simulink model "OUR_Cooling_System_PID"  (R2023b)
settings: Solver=VariableStepAuto  StartTime=0.0  StopTime=10.0  RelTol=1e-3
undefined symbols (not defined in the file): area_air, area_fins, area_primary, cp_air, EM_Spd, EM_Trq, eta_inv, eta_mot, h_tube, HC_min, HC_nom, L_tube, n_tubes, P_nom_pump, rho_air, T_amb, Th_Loss_Inv, Th_Loss_Mot, time, Veh_Spd, vel_air_nom, w_radiator
libraries: fl_lib x29, nesl_utility x16, SimscapeFluids_lib x8, slpidlib x2

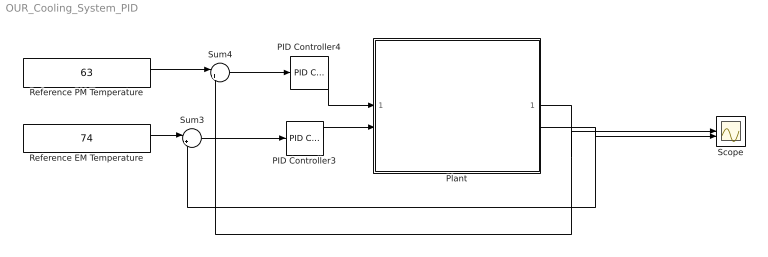
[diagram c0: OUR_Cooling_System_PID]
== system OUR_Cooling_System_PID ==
  PID Controller3 : slpidlib/PID Controller  Controller=PID  Form=Parallel  TimeDomain=Continuous-time  UseExternalTs=off  SampleTime=-1  IntegratorMethod=Forward Euler  FilterMethod=Forward Euler  ControllerParametersSource=internal  P=-0.153121737638524  I=-0.00104451455208141  UseKiTs=off  D=1.82506315689532  N=0.0838994185269757  UseFilter=on  TunerSelectOption=Transfer Function Based (PID Tuner App)  InitialConditionSource=internal  InitialConditionForIntegrator=0  InitialConditionForFilter=0  DifferentiatorICPrevScaledInput=0  ExternalReset=none  TrackingMode=off  Kt=1  LimitOutput=off  SatLimitsSource=internal  UpperSaturationLimit=inf  LowerSaturationLimit=-inf  LinearizeAsGain=on  AntiWindupMode=none  Kb=1  LimitIntegrator=off  UpperIntegratorSaturationLimit=inf  LowerIntegratorSaturationLimit=-inf  POutMin=[]  POutMax=[]  IOutMin=[]  IOutMax=[]  DOutMin=[]  DOutMax=[]  NOutMin=[]  NOutMax=[]  SumOutMin=[]  SumOutMax=[]  SaturationOutMin=[]  SaturationOutMax=[]  PParamMin=[]  PParamMax=[]  IParamMin=[]  IParamMax=[]  DParamMin=[]  DParamMax=[]  NParamMin=[]  NParamMax=[]  KbParamMin=[]  KbParamMax=[]  KtParamMin=[]  KtParamMax=[]  KbOutMin=[]  KbOutMax=[]  KtOutMin=[]  KtOutMax=[]  IntegratorOutMin=[]  IntegratorOutMax=[]  FilterOutMin=[]  FilterOutMax=[]  SumI1OutMin=[]  SumI1OutMax=[]  SumI2OutMin=[]  SumI2OutMax=[]  SumI3OutMin=[]  SumI3OutMax=[]  SumI4OutMin=[]  SumI4OutMax=[]  SumDOutMin=[]  SumDOutMax=[]  DifferentiatorOutMin=[]  DifferentiatorOutMax=[]  FilterDiffOutCoefMin=[]  FilterDiffOutCoefMax=[]  ReciprocalOutMin=[]  ReciprocalOutMax=[]  SumDenOutMin=[]  SumDenOutMax=[]  SumNumOutMin=[]  SumNumOutMax=[]  DivideOutMin=[]  DivideOutMax=[]  UdiffTsProdOutMin=[]  UdiffTsProdOutMax=[]  NTsProdOutMin=[]  NTsProdOutMax=[]  UintegralTsProdOutMin=[]  UintegralTsProdOutMax=[]  UngainTsProdOutMin=[]  UngainTsProdOutMax=[]  ClampingZeroOutDataTypeStr=Inherit: Inherit via back propagation  ClampingZeroOutMin=[]  ClampingZeroOutMax=[]  FilterDenConstantOutDataTypeStr=Inherit: Inherit via back propagation  FilterDenConstantOutMin=[]  FilterDenConstantOutMax=[]  PCopyOutDataTypeStr=Inherit: Inherit via back propagation  PCopyOutMin=[]  PCopyOutMax=[]  NCopyOutDataTypeStr=Inherit: Inherit via back propagation  NCopyOutMin=[]  NCopyOutMax=[]  IntegratorContinuousStateAttributes=''  IntegratorStateMustResolveToSignalObject=off  IntegratorRTWStateStorageClass=Auto  FilterContinuousStateAttributes=''  FilterStateMustResolveToSignalObject=off  FilterRTWStateStorageClass=Auto  ParallelPVariant=InternalParameters  IdealPVariant=Disabled  IVariant=InternalParameters  DVariant=InternalParameters  IntegratorVariant=Continuous  SatVariant=Disabled  AWVariant=Passthrough  PCopyVariant=Disabled  TRVariant=Disabled  FdbkBlocksVariant=Forward  IdealPFdbkVariant=Disabled  SatFdbkVariant=Disabled  DerivativeFilterVariant=ContFilter  NVariant=InternalParameters  NCopyVariant=Disabled  FilterICVariant=InternalICsFilter  IntegratorICVariant=InternalICs  ExternalResetVariant=Disabled  TRSumVariant=Passthrough  SumFdbkVariant=Disabled  SumVariant=Sum_PID  TsampFilterVariant=InternalTs  TsampNgainVariant=Passthrough  TsampIntegralVariant=Disabled_SignalSpec  ExternalSaturationOutDataTypeStr=Inherit: Same as second input
  PID Controller4 : slpidlib/PID Controller  Controller=PID  Form=Parallel  TimeDomain=Continuous-time  UseExternalTs=off  SampleTime=-1  IntegratorMethod=Forward Euler  FilterMethod=Forward Euler  ControllerParametersSource=internal  P=-0.690992720516584  I=-0.00856089702379571  UseKiTs=off  D=21.0718466167788  N=0.0327922242925958  UseFilter=on  TunerSelectOption=Transfer Function Based (PID Tuner App)  InitialConditionSource=internal  InitialConditionForIntegrator=0  InitialConditionForFilter=0  DifferentiatorICPrevScaledInput=0  ExternalReset=none  TrackingMode=off  Kt=1  LimitOutput=off  SatLimitsSource=internal  UpperSaturationLimit=inf  LowerSaturationLimit=-inf  LinearizeAsGain=on  AntiWindupMode=none  Kb=1  LimitIntegrator=off  UpperIntegratorSaturationLimit=inf  LowerIntegratorSaturationLimit=-inf  POutMin=[]  POutMax=[]  IOutMin=[]  IOutMax=[]  DOutMin=[]  DOutMax=[]  NOutMin=[]  NOutMax=[]  SumOutMin=[]  SumOutMax=[]  SaturationOutMin=[]  SaturationOutMax=[]  PParamMin=[]  PParamMax=[]  IParamMin=[]  IParamMax=[]  DParamMin=[]  DParamMax=[]  NParamMin=[]  NParamMax=[]  KbParamMin=[]  KbParamMax=[]  KtParamMin=[]  KtParamMax=[]  KbOutMin=[]  KbOutMax=[]  KtOutMin=[]  KtOutMax=[]  IntegratorOutMin=[]  IntegratorOutMax=[]  FilterOutMin=[]  FilterOutMax=[]  SumI1OutMin=[]  SumI1OutMax=[]  SumI2OutMin=[]  SumI2OutMax=[]  SumI3OutMin=[]  SumI3OutMax=[]  SumI4OutMin=[]  SumI4OutMax=[]  SumDOutMin=[]  SumDOutMax=[]  DifferentiatorOutMin=[]  DifferentiatorOutMax=[]  FilterDiffOutCoefMin=[]  FilterDiffOutCoefMax=[]  ReciprocalOutMin=[]  ReciprocalOutMax=[]  SumDenOutMin=[]  SumDenOutMax=[]  SumNumOutMin=[]  SumNumOutMax=[]  DivideOutMin=[]  DivideOutMax=[]  UdiffTsProdOutMin=[]  UdiffTsProdOutMax=[]  NTsProdOutMin=[]  NTsProdOutMax=[]  UintegralTsProdOutMin=[]  UintegralTsProdOutMax=[]  UngainTsProdOutMin=[]  UngainTsProdOutMax=[]  ClampingZeroOutDataTypeStr=Inherit: Inherit via back propagation  ClampingZeroOutMin=[]  ClampingZeroOutMax=[]  FilterDenConstantOutDataTypeStr=Inherit: Inherit via back propagation  FilterDenConstantOutMin=[]  FilterDenConstantOutMax=[]  PCopyOutDataTypeStr=Inherit: Inherit via back propagation  PCopyOutMin=[]  PCopyOutMax=[]  NCopyOutDataTypeStr=Inherit: Inherit via back propagation  NCopyOutMin=[]  NCopyOutMax=[]  IntegratorContinuousStateAttributes=''  IntegratorStateMustResolveToSignalObject=off  IntegratorRTWStateStorageClass=Auto  FilterContinuousStateAttributes=''  FilterStateMustResolveToSignalObject=off  FilterRTWStateStorageClass=Auto  ParallelPVariant=InternalParameters  IdealPVariant=Disabled  IVariant=InternalParameters  DVariant=InternalParameters  IntegratorVariant=Continuous  SatVariant=Disabled  AWVariant=Passthrough  PCopyVariant=Disabled  TRVariant=Disabled  FdbkBlocksVariant=Forward  IdealPFdbkVariant=Disabled  SatFdbkVariant=Disabled  DerivativeFilterVariant=ContFilter  NVariant=InternalParameters  NCopyVariant=Disabled  FilterICVariant=InternalICsFilter  IntegratorICVariant=InternalICs  ExternalResetVariant=Disabled  TRSumVariant=Passthrough  SumFdbkVariant=Disabled  SumVariant=Sum_PID  TsampFilterVariant=InternalTs  TsampNgainVariant=Passthrough  TsampIntegralVariant=Disabled_SignalSpec  ExternalSaturationOutDataTypeStr=Inherit: Same as second input
  Plant : Subsystem
  Reference EM Temperature : Constant  Value=74
  Reference PM Temperature : Constant  Value=63
  Scope : Scope  NumInputPorts=2
  Sum3 : Sum  Inputs=|+-
  Sum4 : Sum  Inputs=|+-
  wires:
  PID Controller3/1 -> Plant/2(U_pumps)
  Sum3/1 -> PID Controller3/1
  Plant/1(Temperature_out_PM) -> Scope/1, Sum4/2
  Reference PM Temperature/1 -> Sum4/1
  Reference EM Temperature/1 -> Sum3/1
  Sum4/1 -> PID Controller4/1
  Plant/2(Temperature_out_EM) -> Scope/2, Sum3/2
  PID Controller4/1 -> Plant/1(U_fan)

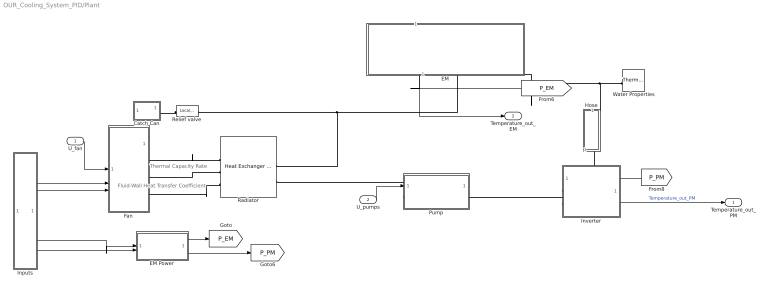
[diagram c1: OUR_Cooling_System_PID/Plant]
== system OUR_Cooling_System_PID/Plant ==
  note: Fluid-Wall Heat Transfer Coefficient
  note: Thermal Capacity Rate
  U_fan : Inport
  U_pumps : Inport  Port=2
  " Water Properties" : SimscapeFluids_lib/Thermal Liquid/Utilities/Thermal Liquid Properties (TL)  fluid_list=fluids.thermal_liquid.utilities.enum.thermal_liquid_fluid_list.water  concentration_param_EG=1  concentration_param_PG=1  c_mass_SW=3.5e-3  c_mass_EG=0.1  c_mass_PG=0.1  c_mass_GL=0.1  c_vol_EG=0.5  c_vol_PG=0.1  beta_const_EG=2.1791 GPa  beta_const_PG=2.1791 GPa  beta_const_GL=2.1791 GPa  p_min_EG=0.01 MPa  p_min_PG=0.01 MPa  p_min_GL=0.01 MPa  p_max_EG=50 MPa  p_max_PG=50 MPa  p_max_GL=50 MPa  p_atm=1 atm  properties_range_check=simscape.enum.assert.action.warn
  Catch Can : Subsystem
  EM : Subsystem
  EM Power : Subsystem
  Fan : Subsystem
  Hose : Subsystem
  Inputs : Subsystem
  Inverter : Subsystem
  Pump : Subsystem
  Radiator : SimscapeFluids_lib/Fluid Network Interfaces/Heat Exchangers/Heat Exchanger (TL)  hex_type=3  shell_num=1  cross_type=4  NTU_TLU=[0.5, 1.0, 2.0, 3.0, 4.0, 5.0]  CR_TLU=[0.0, 0.25, 0.5, 0.75, 1.0]  eff_TLU=[0.3, 0.3, 0.3, 0.3, 0.3; 0.6, 0.55, 0.5, 0.47, 0.43; 0.85, 0.76, 0.68, 0.61, 0.55; 0.94, 0.83, 0.72, 0.65, 0.58; 0.98, 0.86, 0.75, 0.66, 0.58; 0.99, 0.86, 0.75, 0.66, 0.58]  R_wall=0.014/(381*n_tubes*w_radiator*L_tube) K/W  min_flow_area_1=n_tubes*(w_radiator*h_tube) m^2  Dh_press_1=4*(w_radiator*h_tube)/(2 * (w_radiator+h_tube)) m  liquid_volume_1=n_tubes*(w_radiator*h_tube)*L_tube m^3  Re_lam_1=2000  Re_tur_1=4000  pressure_loss_spec_1=2  pressure_loss_coeff_1=15  length_press_1=L_tube m  length_add_1=0.1 m  roughness_1=15e-6 m  Re_friction_TLU_1=[400.0, 1000.0, 1500.0, 3000.0, 4000.0, 6000.0, 10000.0, 20000.0, 40000.0, 60000.0, 100000.0, 100000000.0]  friction_factor_TLU_1=[0.264, 0.112, 0.071, 0.0417, 0.0387, 0.0268, 0.025, 0.0232, 0.0226, 0.022, 0.0214, 0.0214]  shape_factor_1=64  Re_Euler_TLU_1=[50.0, 500.0, 1000.0, 2000.0]  Euler_TLU_1=[4.4505, 0.6864, 0.4791, 0.3755]  heat_transfer_spec_1=2  heat_transfer_area_1=n_tubes*2*(L_tube*w_radiator+L_tube*h_tube) m^2  heat_coeff_1=2000 W/(m^2 * K)  length_heat_1=L_tube m  Nu_lam_1=3.66  Re_Colburn_TLU_1=[100.0, 150.0, 1000.0]  Colburn_factor_TLU_1=[0.019, 0.013, 0.002]  Re_Nu_TLU_1=[100.0, 150.0, 1000.0]  Pr_Nu_TLU_1=[1.0, 10.0]  Nu_TLU_1=[3.72, 4.21; 3.75, 4.44; 4.21, 7.15]  fouling_factor_1=0 m^2*K/W  min_heat_coeff_1=5 W/(m^2 * K)  heat_transfer_area_2=area_primary+area_fins m^2  fouling_factor_2=0 m^2*K/W  min_heat_coeff_2=0.01 W/(m^2 * K)  dynamic_compressibility_1=1  T0_1=293.15 K  p0_1=0.101325 MPa  mdot1_TLU=[.1, .2] kg/s  mdot2_TLU=[.2, .3] kg/s  SD_TLU=[35, 35; 50, 50] kW/K  Q_check=1  mdot_dp_TLU_1=[.1, .2] kg/s  p_diff_TLU_1=[.003, .005] MPa  T_ref_in_1=293.15 K  p_ref_in_1=0.101325 MPa  mdot_threshold_1=1e-3 kg/s  area_1=0.01 m^2
  Relief valve : fl_lib/Thermal Liquid/Elements/Local Restriction (TL)  restriction_type=foundation.enum.restriction_type.fixed  restriction_area=pi*0.005^2 m^2  min_area=1e-10 m^2  max_area=0.005 m^2  area=pi*0.01^2 m^2  Cd=0.7  Re_c=12  pressure_recovery=1
  Temperature_out_PM : Outport
  Temperature_out_EM : Outport  Port=2
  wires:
  Inputs/3(EM_torque) -> EM Power/1(EM_torque)
  EM Power/2(P_PM) -> [P_PM]
  [P_PM] -> Inverter/1(Invert_Power)
  Inputs/4(EM_speed) -> EM Power/2(EM_speed)
  [P_EM] -> EM/1(EM_Power)
  EM Power/1(P_EM) -> [P_EM]
  Inputs/1(Veh_speed) -> Fan/2(V)
  Inputs/2(T_air) -> Fan/3(Tair)
  Inverter/1(T_PM_Out) -> Temperature_out_PM/1  "Temperature_out_PM"
  U_fan/1 -> Fan/1(U_fan)
  U_pumps/1 -> Pump/1(U_pump)
  EM/1(T_Out_EM) -> Temperature_out_EM/1
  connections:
  Relief valve/LConn1 -- Catch Can/RConn1
  Relief valve/RConn1 -- Radiator/LConn1 -- EM/LConn1
  Radiator/RConn1 -- Fan/RConn1
  Pump/LConn1 -- Radiator/LConn2
  Hose/LConn1 -- Inverter/LConn2
  Radiator/RConn3 -- Fan/RConn3
  Radiator/RConn2 -- Fan/RConn2
  " Water Properties"/RConn1 -- EM/RConn1 -- Hose/RConn1
  Inverter/LConn1 -- Pump/RConn1

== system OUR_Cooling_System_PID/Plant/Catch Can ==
  Catch Can : SimscapeFluids_lib/Thermal Liquid/Tanks & Accumulators/Gas-Charged Accumulator (TL)  capacity=0.005 m^3  dead_volume=1e-5 m^3  p_precharge_gauge=0 MPa  k_sh=1.4  area=pi*0.01^2 m^2  stiff_coeff=1e6 MPa/m^3  damping_coeff=1e6 s*MPa/m^6  liquid_volume_specify=on  liquid_volume_priority=High  liquid_volume=1e-6 m^3  liquid_volume_nominal_specify=off  liquid_volume_nominal_unit=m^3  liquid_volume_nominal_value=1  liquid_mass_specify=off  liquid_mass_priority=None  liquid_mass=5 kg  liquid_mass_nominal_specify=off  liquid_mass_nominal_unit=kg  liquid_mass_nominal_value=1  p_I_specify=off  p_I_priority=High  p_I=0.101325 MPa  p_I_nominal_specify=off  p_I_nominal_unit=MPa  p_I_nominal_value=1  T_I_specify=on  T_I_priority=High  T_I=303.15 K  T_I_nominal_specify=off  T_I_nominal_unit=K  T_I_nominal_value=1
  Perfect Insulator2 : fl_lib/Thermal/Thermal Elements/Perfect Insulator  T_specify=off  T_priority=None  T=0 K  T_nominal_specify=off  T_nominal_unit=K  T_nominal_value=1
  Connection Port : PMIOPort  Side=Right
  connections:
  Connection Port/RConn1 -- Catch Can/RConn1
  Perfect Insulator2/LConn1 -- Catch Can/RConn2

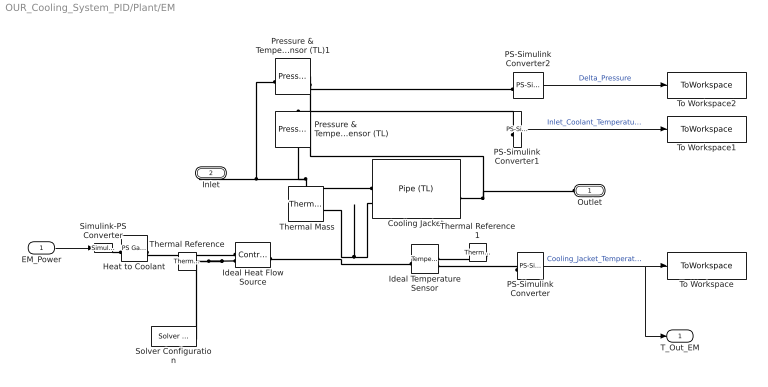
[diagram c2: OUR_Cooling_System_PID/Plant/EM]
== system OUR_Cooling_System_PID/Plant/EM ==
  EM_Power : Inport
  " Thermal Mass" : fl_lib/Thermal/Thermal Elements/Thermal Mass  mass_type=foundation.enum.constant_variable.constant  mass=46.7 kg  sp_heat=447 J/kg/K  mass_min=1e-6 kg  num_ports=foundation.enum.numPorts2.one  m_specify=off  m_priority=High  m=1 kg  m_nominal_specify=off  m_nominal_unit=kg  m_nominal_value=1  T_specify=on  T_priority=High  T=30 degC  T_nominal_specify=off  T_nominal_unit=K  T_nominal_value=1  Q_specify=off  Q_priority=High  Q=0 J/s  Q_nominal_specify=off  Q_nominal_unit=J/s  Q_nominal_value=1
  Cooling Jacket : SimscapeFluids_lib/Thermal Liquid/Pipes & Fittings/Pipe (TL)  dynamic_compressibility=simscape.enum.onoff.on  inertia=simscape.enum.onoff.off  num_segments=1  pipe_length=0.2 m  cross_section_geometry=fluids.thermal_liquid.pipes_fittings.enum.CrossSectionGeometry.Custom  pipe_diameter=0.1 m  pipe_inner_diameter=0.05 m  pipe_outer_diameter=0.1 m  pipe_width=0.1 m  pipe_height=0.1 m  pipe_major_axis=0.1 m  pipe_minor_axis=0.05 m  pipe_side=0.1 m  pipe_angle=30 deg  area=pi*0.01^2 m^2  Dh=0.005 m  elevation_spec=foundation.enum.constant_variable.constant  elevation_gain=0 m  gravity_spec=foundation.enum.constant_variable.constant  g=9.81 m/s^2  pressure_loss_spec=fluids.thermal_liquid.pipes_fittings.enum.PressureLossSpec.Nominal  local_pressure_loss_spec=fluids.thermal_liquid.pipes_fittings.enum.LocalLossSpec.AggregateLength  length_add=1 m  loss_coefficient=0.1  roughness_spec=fluids.thermal_liquid.pipes_fittings.enum.RoughnessSpec.Custom  roughness=1.5e-5 m  Re_friction_TLU=[ 400 1000 1.5e+3 3e+3 4e+3 6e+3 1e+4 2e+4 4e+4 6e+4 1e+5 1e+8 ]  friction_factor_TLU=[ 0.264 0.112 0.07099999999999999 0.0417 0.0387 0.0268 0.025 0.0232 0.0226 0.022 0.0214 0.0214 ]  Re_lam=2e+3  Re_tur=4e+3  shape_factor=64  mdot_nominal=[ 0.1 0.2 ] kg/s  p_diff_nominal=[ 12 12 ] kPa  mdot_threshold=1e-6 kg/s  wall_spec=fluids.thermal_liquid.pipes_fittings.enum.wall_spec.rigid  vol_expansion_spec=fluids.thermal_liquid.pipes_fittings.enum.VolumeExpansionSpec.Diameter  area_pressure_gain=1e-6 m^2/MPa  static_pressure_TLU=[.1, 1] MPa  area_pressure_gain_TLU=[1e-05, 1.1e-05] m^2  material_behavior_spec=fluids.thermal_liquid.pipes_fittings.enum.PipeMaterialBehavior.Linear  diameter_pressure_gain=1.2e-6 m/MPa  wall_thickness=0.05 m  elastic_modulus=69 GPa  stress_TLU=[276, 310] MPa  strain_TLU=[.004, .02]  stress_assert_action=simscape.enum.assert.action.none  stress_max=400 MPa  poisson_ratio=0.33  wall_time_constant=0.01 s  thermal_expansion=false  alpha_L_wall=24 um/(deltaK*m)  thermal_expansion_Tref=293.15 K  heat_transfer_spec=fluids.thermal_liquid.pipes_fittings.enum.HeatTransferSpec.TabulatedNusselt  mdot_nominal_heat=[ 0.1 1 ] kg/s  T_in_nominal=[ 293.15 293.15 ] K  T_out_nominal=[ 300 300 ] K  p_in_nominal_heat=[ 0.101325 0.101325 ] MPa  T_wall_nominal=[ 303.15 303.15 ] K  a_coeff=0.023  b_Re_power=0.8  c_Pr_power=0.4  Nu_lam=3.66  Re_Colburn_TLU=[ 100 150 1000 ]  Colburn_factor_TLU=[ 0.019 0.013 0.002 ]  Re_Nu_TLU=Re_TLU  Pr_Nu_TLU=Pr_TLU  Nu_TLU=Nu_TLU  p0_vec=0.101325 MPa  T0_vec=303.15 K  mdot0=0.1 kg/s
  Heat to Coolant : fl_lib/Physical Signals/Functions/PS Gain  gain=Th_Loss_Mot
  Ideal Heat Flow Source : fl_lib/Thermal/Thermal Sources/Controlled Heat Flow Rate Source
  Ideal Temperature Sensor : fl_lib/Thermal/Thermal Sensors/Temperature Sensor  temperature_measure=foundation.enum.MeasurementReference.difference
  PS-Simulink Converter : nesl_utility/PS-Simulink Converter  PhysicalDomain=network_engine_domain  SubClassName=ps_output  LeftPortType=input  RightPortType=output  PseudoPeriodic=off  Frequencies=[]  VectorFormat=1-D array  Unit=degC  AffineConversion=on
  PS-Simulink Converter1 : nesl_utility/PS-Simulink Converter  PhysicalDomain=network_engine_domain  SubClassName=ps_output  LeftPortType=input  RightPortType=output  PseudoPeriodic=off  Frequencies=[]  VectorFormat=1-D array  Unit=degC  AffineConversion=on
  PS-Simulink Converter2 : nesl_utility/PS-Simulink Converter  PhysicalDomain=network_engine_domain  SubClassName=ps_output  LeftPortType=input  RightPortType=output  PseudoPeriodic=off  Frequencies=[]  VectorFormat=1-D array  Unit=Pa  AffineConversion=on
  Pressure & Temperature Sensor (TL) : fl_lib/Thermal Liquid/Sensors/Pressure & Temperature Sensor (TL)  reference=foundation.enum.MeasurementReference.absolute  pressure=false  pressure_spec=foundation.enum.PressureMeasementSpec.Absolute  temperature=true
  Pressure & Temperature Sensor (TL)1 : fl_lib/Thermal Liquid/Sensors/Pressure & Temperature Sensor (TL)  reference=foundation.enum.MeasurementReference.difference  pressure=true  pressure_spec=foundation.enum.PressureMeasementSpec.Absolute  temperature=false
  Simulink-PS Converter : nesl_utility/Simulink-PS Converter  PhysicalDomain=network_engine_domain  SubClassName=ps_input  LeftPortType=input  RightPortType=output  PseudoPeriodic=off  Frequencies=[]  NoiseDistribution=none  NoiseParameters=[]  Unit=W  AffineConversion=off  FilteringAndDerivatives=provide  SimscapeFilterOrder=1  InputFilterTimeConstant=0.001  UdotUserProvided=0
  Solver Configuration : nesl_utility/Solver Configuration  PhysicalDomain=network_engine_domain  SubClassName=solver  LeftPortType=input  RightPortType=generic  Tones=[]  Harmonics=[]  SimulateNoise=off  Profile=off  UseLocalSampling=off  EnableSwitchedLinearOptims=on  FrequencyDomain=off  UseCCode=off  RelTol=0.001  AbsTol=1e-06  MinStep=1e-09  ToWorkspace=off  RevertToSquareIcSolve=off  NumHomotopyIterations=100  PhasorMode=off  PhasorModeNumHarmonics=1  ConsistencySolver=NEWTON_XTOL_AFTER_FTOL  IndexReductionMethod=DerivativeReplacement  DoDC=off  ResidualTolerance=1e-9  ConsistencyTolSource=GLOBAL  ConsistencyAbsTol=0.001  ConsistencyRelTol=0.001  ConsistencyTolFactor=0.001  UseLocalSolver=off  LocalSolverChoice=NE_BACKWARD_EULER_ADVANCER  ResolveIndetEquations=on  FunctionEvalNumThread=1  LocalSolverSampleTime=1  DoFixedCost=off  MaxNonlinIter=3  MaxModeIter=2  ComputeImpulses=off  ImpulseIterations=2  LinearAlgebra=auto  LinearAlgebraNumThread=0  EquationFormulation=NE_TIME_EF  DelaysMemoryBudget=1024  AutomaticFiltering=on  FilteringTimeConstant=0.001  PartitionStorageMethod=AS_NEEDED  PartitionMemoryBudget=1024  PartitionMethod=FAST  MultibodyUseLocalSolver=off  MultibodyLocalSolverChoice=ODE1  MultibodyLocalSolverSampleTime=0.001
  Thermal Reference : fl_lib/Thermal/Thermal Elements/Thermal Reference
  Thermal Reference1 : fl_lib/Thermal/Thermal Elements/Thermal Reference
  To Workspace : ToWorkspace  VariableName=T_EM  SaveFormat=Timeseries  SampleTime=-1
  To Workspace1 : ToWorkspace  VariableName=TC_EM_IN  SaveFormat=Timeseries  SampleTime=-1
  To Workspace2 : ToWorkspace  VariableName=deltaP_EM  SaveFormat=Timeseries  SampleTime=-1
  Outlet : PMIOPort  Side=Left
  Inlet : PMIOPort  Port=2  Side=Right
  T_Out_EM : Outport
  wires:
  EM_Power/1 -> Simulink-PS Converter/1
  PS-Simulink Converter/1 -> T_Out_EM/1, To Workspace/1  "Cooling_Jacket_Temperature"
  PS-Simulink Converter2/1 -> To Workspace2/1  "Delta_Pressure"
  PS-Simulink Converter1/1 -> To Workspace1/1  "Inlet_Coolant_Temperature"
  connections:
  Ideal Heat Flow Source/RConn2 -- Thermal Reference/LConn1 -- Solver Configuration/RConn1
  Heat to Coolant/RConn1 -- Ideal Heat Flow Source/RConn1
  Cooling Jacket/RConn1 -- Outlet/RConn1 -- Pressure & Temperature Sensor (TL)1/RConn1
  Simulink-PS Converter/RConn1 -- Heat to Coolant/LConn1
  Pressure & Temperature Sensor (TL)1/LConn1 -- Pressure & Temperature Sensor (TL)/LConn1 -- Cooling Jacket/LConn1 -- Inlet/RConn1
  PS-Simulink Converter/LConn1 -- Ideal Temperature Sensor/RConn2
  Ideal Heat Flow Source/LConn1 -- Ideal Temperature Sensor/LConn1 -- " Thermal Mass"/LConn1 -- Cooling Jacket/LConn2
  Thermal Reference1/LConn1 -- Ideal Temperature Sensor/RConn1
  Pressure & Temperature Sensor (TL)1/RConn2 -- PS-Simulink Converter2/LConn1
  PS-Simulink Converter1/LConn1 -- Pressure & Temperature Sensor (TL)/RConn1

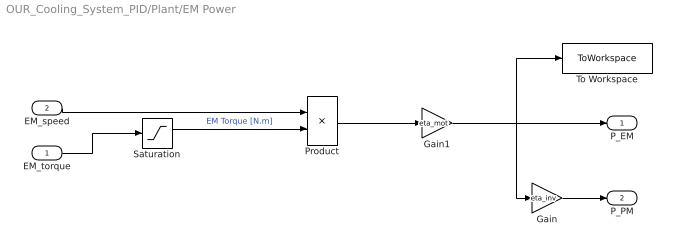
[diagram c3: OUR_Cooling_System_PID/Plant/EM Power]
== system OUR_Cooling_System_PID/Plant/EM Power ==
  EM_torque : Inport
  EM_speed : Inport  Port=2
  Gain : Gain  Gain=eta_inv
  Gain1 : Gain  Gain=eta_mot
  Product : Product
  Saturation : Saturate  UpperLimit=inf  LowerLimit=0
  To Workspace : ToWorkspace  VariableName=P_EM  SaveFormat=Timeseries  SampleTime=-1
  P_EM : Outport  VectorParamsAs1DForOutWhenUnconnected=off
  P_PM : Outport  Port=2
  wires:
  Saturation/1 -> Product/2  "EM Torque [N.m]"
  EM_torque/1 -> Saturation/1
  Product/1 -> Gain1/1
  EM_speed/1 -> Product/1
  Gain/1 -> P_PM/1
  Gain1/1 -> To Workspace/1, P_EM/1, Gain/1

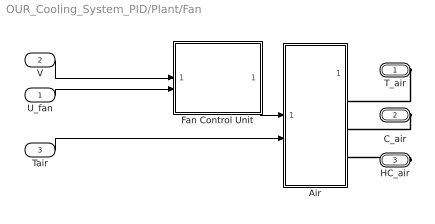
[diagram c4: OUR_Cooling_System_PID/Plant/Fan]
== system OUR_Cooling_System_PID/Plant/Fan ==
  U_fan : Inport
  V : Inport  Port=2
  Tair : Inport  Port=3
  Air : Subsystem
  Fan Control Unit : Subsystem
  T_air : PMIOPort  Side=Right
  C_air : PMIOPort  Port=2  Side=Right
  HC_air : PMIOPort  Port=3  Side=Right
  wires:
  Tair/1 -> Air/2(T_air)
  V/1 -> Fan Control Unit/1(Veh_speed)
  Fan Control Unit/1(V_air (m/s)) -> Air/1(V_air)
  U_fan/1 -> Fan Control Unit/2(U_fan)
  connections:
  T_air/RConn1 -- Air/RConn1
  C_air/RConn1 -- Air/RConn2
  HC_air/RConn1 -- Air/RConn3

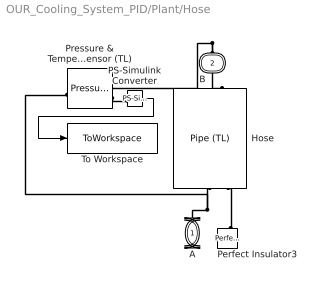
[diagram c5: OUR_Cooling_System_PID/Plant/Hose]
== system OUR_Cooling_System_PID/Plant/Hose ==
  Hose : SimscapeFluids_lib/Thermal Liquid/Pipes & Fittings/Pipe (TL)  dynamic_compressibility=simscape.enum.onoff.on  inertia=simscape.enum.onoff.off  num_segments=1  pipe_length=0.7 m  cross_section_geometry=fluids.thermal_liquid.pipes_fittings.enum.CrossSectionGeometry.Custom  pipe_diameter=0.1 m  pipe_inner_diameter=0.05 m  pipe_outer_diameter=0.1 m  pipe_width=0.1 m  pipe_height=0.1 m  pipe_major_axis=0.1 m  pipe_minor_axis=0.05 m  pipe_side=0.1 m  pipe_angle=30 deg  area=pi*0.005^2 m^2  Dh=0.05 m  elevation_spec=foundation.enum.constant_variable.constant  elevation_gain=0 m  gravity_spec=foundation.enum.constant_variable.constant  g=9.81 m/s^2  pressure_loss_spec=fluids.thermal_liquid.pipes_fittings.enum.PressureLossSpec.Haaland  local_pressure_loss_spec=fluids.thermal_liquid.pipes_fittings.enum.LocalLossSpec.AggregateLength  length_add=5 m  loss_coefficient=0.1  roughness_spec=fluids.thermal_liquid.pipes_fittings.enum.RoughnessSpec.Custom  roughness=1.5e-5 m  Re_friction_TLU=[ 400 1000 1.5e+3 3e+3 4e+3 6e+3 1e+4 2e+4 4e+4 6e+4 1e+5 1e+8 ]  friction_factor_TLU=[ 0.264 0.112 0.07099999999999999 0.0417 0.0387 0.0268 0.025 0.0232 0.0226 0.022 0.0214 0.0214 ]  Re_lam=2e+3  Re_tur=4e+3  shape_factor=64  mdot_nominal=[ 0.1 1 ] kg/s  p_diff_nominal=[ 0.001 0.01 ] MPa  mdot_threshold=1e-6 kg/s  wall_spec=fluids.thermal_liquid.pipes_fittings.enum.wall_spec.flexible  vol_expansion_spec=fluids.thermal_liquid.pipes_fittings.enum.VolumeExpansionSpec.Diameter  area_pressure_gain=1e-6 m^2/MPa  static_pressure_TLU=[.1, 1] MPa  area_pressure_gain_TLU=[1e-05, 1.1e-05] m^2  material_behavior_spec=fluids.thermal_liquid.pipes_fittings.enum.PipeMaterialBehavior.Linear  diameter_pressure_gain=1.2e-6 m/MPa  wall_thickness=0.05 m  elastic_modulus=69 GPa  stress_TLU=[276, 310] MPa  strain_TLU=[.004, .02]  stress_assert_action=simscape.enum.assert.action.none  stress_max=400 MPa  poisson_ratio=0.33  wall_time_constant=0.01 s  thermal_expansion=false  alpha_L_wall=24 um/(deltaK*m)  thermal_expansion_Tref=293.15 K  heat_transfer_spec=fluids.thermal_liquid.pipes_fittings.enum.HeatTransferSpec.Gnielinski  mdot_nominal_heat=[ 0.1 1 ] kg/s  T_in_nominal=[ 293.15 293.15 ] K  T_out_nominal=[ 300 300 ] K  p_in_nominal_heat=[ 0.101325 0.101325 ] MPa  T_wall_nominal=[ 303.15 303.15 ] K  a_coeff=0.023  b_Re_power=0.8  c_Pr_power=0.4  Nu_lam=3.66  Re_Colburn_TLU=[ 100 150 1000 ]  Colburn_factor_TLU=[ 0.019 0.013 0.002 ]  Re_Nu_TLU=[ 100 150 1000 ]  Pr_Nu_TLU=[ 1 10 ]  Nu_TLU=[ 3.72 4.21; 3.75 4.44; 4.21 7.15 ]  p0_vec=0.101325 MPa  T0_vec=303.15 K  mdot0=0.1 kg/s
  PS-Simulink Converter : nesl_utility/PS-Simulink Converter  PhysicalDomain=network_engine_domain  SubClassName=ps_output  LeftPortType=input  RightPortType=output  PseudoPeriodic=off  Frequencies=[]  VectorFormat=inherit  Unit=inherit  AffineConversion=off
  Perfect Insulator3 : fl_lib/Thermal/Thermal Elements/Perfect Insulator  T_specify=off  T_priority=None  T=0 K  T_nominal_specify=off  T_nominal_unit=K  T_nominal_value=1
  Pressure & Temperature Sensor (TL) : fl_lib/Thermal Liquid/Sensors/Pressure & Temperature Sensor (TL)  reference=foundation.enum.MeasurementReference.difference  pressure=true  pressure_spec=foundation.enum.PressureMeasementSpec.Absolute  temperature=false
  To Workspace : ToWorkspace  VariableName=simout  SaveFormat=Timeseries  SampleTime=-1
  A : PMIOPort  Side=Left
  B : PMIOPort  Port=2  Side=Right
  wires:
  PS-Simulink Converter/1 -> To Workspace/1
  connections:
  Perfect Insulator3/LConn1 -- Hose/LConn2
  Pressure & Temperature Sensor (TL)/LConn1 -- A/RConn1 -- Hose/LConn1
  B/RConn1 -- Pressure & Temperature Sensor (TL)/RConn1 -- Hose/RConn1
  Pressure & Temperature Sensor (TL)/RConn2 -- PS-Simulink Converter/LConn1

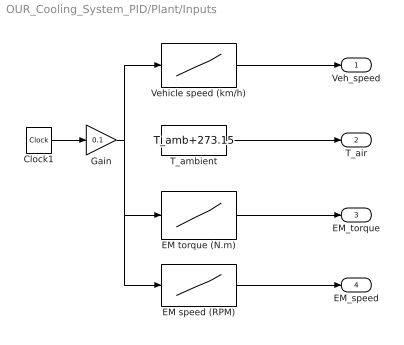
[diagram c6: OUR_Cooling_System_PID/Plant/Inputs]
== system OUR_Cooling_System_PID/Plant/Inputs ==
  Clock1 : Clock
  EM speed (RPM) : Lookup  InputValues=time  Table=EM_Spd  LookUpMeth=Interpolation-Use End Values
  EM torque (N.m) : Lookup  InputValues=time  Table=EM_Trq  LookUpMeth=Interpolation-Use End Values
  Gain : Gain  Gain=0.1
  T_ambient : Constant  Value=T_amb+273.15
  Vehicle speed (km/h) : Lookup  InputValues=time  Table=Veh_Spd  LookUpMeth=Interpolation-Use End Values
  Veh_speed : Outport  VectorParamsAs1DForOutWhenUnconnected=off
  T_air : Outport  Port=2  VectorParamsAs1DForOutWhenUnconnected=off
  EM_torque : Outport  Port=3  VectorParamsAs1DForOutWhenUnconnected=off
  EM_speed : Outport  Port=4  VectorParamsAs1DForOutWhenUnconnected=off
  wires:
  Gain/1 -> EM speed (RPM)/1, EM torque (N.m)/1, Vehicle speed (km/h)/1
  EM torque (N.m)/1 -> EM_torque/1
  Clock1/1 -> Gain/1
  EM speed (RPM)/1 -> EM_speed/1
  Vehicle speed (km/h)/1 -> Veh_speed/1
  T_ambient/1 -> T_air/1

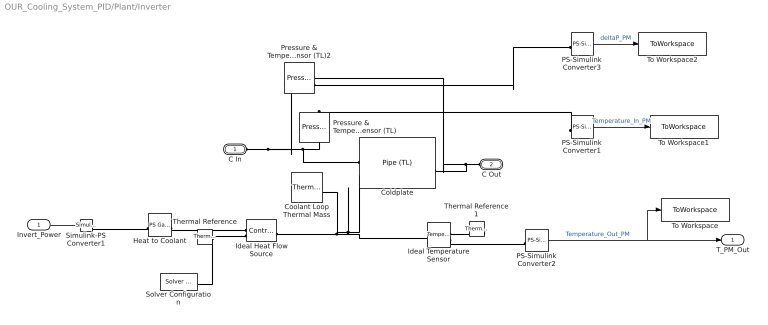
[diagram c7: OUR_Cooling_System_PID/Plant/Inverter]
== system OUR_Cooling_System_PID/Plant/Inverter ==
  Invert_Power : Inport
  Coldplate : SimscapeFluids_lib/Thermal Liquid/Pipes & Fittings/Pipe (TL)  dynamic_compressibility=simscape.enum.onoff.on  inertia=simscape.enum.onoff.off  num_segments=3  pipe_length=PM_Pipe_Length m  cross_section_geometry=fluids.thermal_liquid.pipes_fittings.enum.CrossSectionGeometry.Circular  pipe_diameter=PM_Pipe_Diameter m  pipe_inner_diameter=0.05 m  pipe_outer_diameter=0.1 m  pipe_width=0.1 m  pipe_height=0.1 m  pipe_major_axis=0.1 m  pipe_minor_axis=0.05 m  pipe_side=0.1 m  pipe_angle=30 deg  area=pi*0.01^2 m^2  Dh=0.005 m  elevation_spec=foundation.enum.constant_variable.constant  elevation_gain=0 m  gravity_spec=foundation.enum.constant_variable.constant  g=9.81 m/s^2  pressure_loss_spec=fluids.thermal_liquid.pipes_fittings.enum.PressureLossSpec.Nominal  local_pressure_loss_spec=fluids.thermal_liquid.pipes_fittings.enum.LocalLossSpec.AggregateLength  length_add=1 m  loss_coefficient=0.1  roughness_spec=fluids.thermal_liquid.pipes_fittings.enum.RoughnessSpec.Custom  roughness=1.5e-5 m  Re_friction_TLU=[ 400 1000 1.5e+3 3e+3 4e+3 6e+3 1e+4 2e+4 4e+4 6e+4 1e+5 1e+8 ]  friction_factor_TLU=[ 0.264 0.112 0.07099999999999999 0.0417 0.0387 0.0268 0.025 0.0232 0.0226 0.022 0.0214 0.0214 ]  Re_lam=2e+3  Re_tur=4e+3  shape_factor=64  mdot_nominal=[0.1 0.2] kg/s  p_diff_nominal=[4 4] kPa  mdot_threshold=1e-6 kg/s  wall_spec=fluids.thermal_liquid.pipes_fittings.enum.wall_spec.rigid  vol_expansion_spec=fluids.thermal_liquid.pipes_fittings.enum.VolumeExpansionSpec.Diameter  area_pressure_gain=1e-6 m^2/MPa  static_pressure_TLU=[.1, 1] MPa  area_pressure_gain_TLU=[1e-05, 1.1e-05] m^2  material_behavior_spec=fluids.thermal_liquid.pipes_fittings.enum.PipeMaterialBehavior.Linear  diameter_pressure_gain=1.2e-6 m/MPa  wall_thickness=0.05 m  elastic_modulus=69 GPa  stress_TLU=[276, 310] MPa  strain_TLU=[.004, .02]  stress_assert_action=simscape.enum.assert.action.none  stress_max=400 MPa  poisson_ratio=0.33  wall_time_constant=0.01 s  thermal_expansion=false  alpha_L_wall=24 um/(deltaK*m)  thermal_expansion_Tref=293.15 K  heat_transfer_spec=fluids.thermal_liquid.pipes_fittings.enum.HeatTransferSpec.TabulatedNusselt  mdot_nominal_heat=[ 0.1 1 ] kg/s  T_in_nominal=[ 293.15 293.15 ] K  T_out_nominal=[ 300 300 ] K  p_in_nominal_heat=[ 0.101325 0.101325 ] MPa  T_wall_nominal=[ 303.15 303.15 ] K  a_coeff=0.023  b_Re_power=0.8  c_Pr_power=0.4  Nu_lam=3.66  Re_Colburn_TLU=[ 100 150 1000 ]  Colburn_factor_TLU=[ 0.019 0.013 0.002 ]  Re_Nu_TLU=Re_TLU  Pr_Nu_TLU=Pr_TLU  Nu_TLU=Nu_TLU  p0_vec=0.101325 MPa  T0_vec=303.15 K  mdot0=0.1 kg/s
  Coolant Loop Thermal Mass : fl_lib/Thermal/Thermal Elements/Thermal Mass  mass_type=foundation.enum.constant_variable.constant  mass=40 kg  sp_heat=400 J/kg/K  mass_min=1e-6 kg  num_ports=foundation.enum.numPorts2.one  m_specify=off  m_priority=High  m=1 kg  m_nominal_specify=off  m_nominal_unit=kg  m_nominal_value=1  T_specify=on  T_priority=High  T=30 degC  T_nominal_specify=off  T_nominal_unit=K  T_nominal_value=1  Q_specify=off  Q_priority=High  Q=0 J/s  Q_nominal_specify=off  Q_nominal_unit=J/s  Q_nominal_value=1
  Heat to Coolant : fl_lib/Physical Signals/Functions/PS Gain  gain=Th_Loss_Inv
  Ideal Heat Flow Source : fl_lib/Thermal/Thermal Sources/Controlled Heat Flow Rate Source
  Ideal Temperature Sensor : fl_lib/Thermal/Thermal Sensors/Temperature Sensor  temperature_measure=foundation.enum.MeasurementReference.difference
  PS-Simulink Converter1 : nesl_utility/PS-Simulink Converter  PhysicalDomain=network_engine_domain  SubClassName=ps_output  LeftPortType=input  RightPortType=output  PseudoPeriodic=off  Frequencies=[]  VectorFormat=1-D array  Unit=degC  AffineConversion=on
  PS-Simulink Converter2 : nesl_utility/PS-Simulink Converter  PhysicalDomain=network_engine_domain  SubClassName=ps_output  LeftPortType=input  RightPortType=output  PseudoPeriodic=off  Frequencies=[]  VectorFormat=1-D array  Unit=degC  AffineConversion=on
  PS-Simulink Converter3 : nesl_utility/PS-Simulink Converter  PhysicalDomain=network_engine_domain  SubClassName=ps_output  LeftPortType=input  RightPortType=output  PseudoPeriodic=off  Frequencies=[]  VectorFormat=1-D array  Unit=Pa  AffineConversion=on
  Pressure & Temperature Sensor (TL) : fl_lib/Thermal Liquid/Sensors/Pressure & Temperature Sensor (TL)  reference=foundation.enum.MeasurementReference.absolute  pressure=false  pressure_spec=foundation.enum.PressureMeasementSpec.Absolute  temperature=true
  Pressure & Temperature Sensor (TL)2 : fl_lib/Thermal Liquid/Sensors/Pressure & Temperature Sensor (TL)  reference=foundation.enum.MeasurementReference.difference  pressure=true  pressure_spec=foundation.enum.PressureMeasementSpec.Absolute  temperature=false
  Simulink-PS Converter1 : nesl_utility/Simulink-PS Converter  PhysicalDomain=network_engine_domain  SubClassName=ps_input  LeftPortType=input  RightPortType=output  PseudoPeriodic=off  Frequencies=[]  NoiseDistribution=none  NoiseParameters=[]  Unit=1  AffineConversion=off  FilteringAndDerivatives=provide  SimscapeFilterOrder=1  InputFilterTimeConstant=0.001  UdotUserProvided=0
  Solver Configuration : nesl_utility/Solver Configuration  PhysicalDomain=network_engine_domain  SubClassName=solver  LeftPortType=input  RightPortType=generic  Tones=[]  Harmonics=[]  SimulateNoise=off  Profile=off  UseLocalSampling=off  EnableSwitchedLinearOptims=on  FrequencyDomain=off  UseCCode=off  RelTol=0.001  AbsTol=1e-06  MinStep=1e-09  ToWorkspace=off  RevertToSquareIcSolve=off  NumHomotopyIterations=100  PhasorMode=off  PhasorModeNumHarmonics=1  ConsistencySolver=NEWTON_XTOL_AFTER_FTOL  IndexReductionMethod=DerivativeReplacement  DoDC=off  ResidualTolerance=1e-9  ConsistencyTolSource=GLOBAL  ConsistencyAbsTol=0.001  ConsistencyRelTol=0.001  ConsistencyTolFactor=0.001  UseLocalSolver=off  LocalSolverChoice=NE_BACKWARD_EULER_ADVANCER  ResolveIndetEquations=on  FunctionEvalNumThread=1  LocalSolverSampleTime=1  DoFixedCost=off  MaxNonlinIter=3  MaxModeIter=2  ComputeImpulses=off  ImpulseIterations=2  LinearAlgebra=auto  LinearAlgebraNumThread=0  EquationFormulation=NE_TIME_EF  DelaysMemoryBudget=1024  AutomaticFiltering=on  FilteringTimeConstant=0.001  PartitionStorageMethod=AS_NEEDED  PartitionMemoryBudget=1024  PartitionMethod=FAST  MultibodyUseLocalSolver=off  MultibodyLocalSolverChoice=ODE1  MultibodyLocalSolverSampleTime=0.001
  Thermal Reference : fl_lib/Thermal/Thermal Elements/Thermal Reference
  Thermal Reference1 : fl_lib/Thermal/Thermal Elements/Thermal Reference
  To Workspace : ToWorkspace  VariableName=T_PM_OUT  SaveFormat=Timeseries  SampleTime=-1
  To Workspace1 : ToWorkspace  VariableName=T_PM_IN  SaveFormat=Timeseries  SampleTime=-1
  To Workspace2 : ToWorkspace  VariableName=deltaP_PM  SaveFormat=Timeseries  SampleTime=-1
  C In : PMIOPort  Side=Left
  C Out : PMIOPort  Port=2  Side=Left
  T_PM_Out : Outport
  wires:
  Invert_Power/1 -> Simulink-PS Converter1/1
  PS-Simulink Converter2/1 -> To Workspace/1, T_PM_Out/1  "Temperature_Out_PM"
  PS-Simulink Converter1/1 -> To Workspace1/1  "Temperature_In_PM"
  PS-Simulink Converter3/1 -> To Workspace2/1  "deltaP_PM"
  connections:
  C Out/RConn1 -- Pressure & Temperature Sensor (TL)2/RConn1 -- Coldplate/RConn1
  Ideal Heat Flow Source/LConn1 -- Ideal Temperature Sensor/LConn1 -- Coolant Loop Thermal Mass/LConn1 -- Coldplate/LConn2
  Simulink-PS Converter1/RConn1 -- Heat to Coolant/LConn1
  Heat to Coolant/RConn1 -- Ideal Heat Flow Source/RConn1
  Thermal Reference/LConn1 -- Solver Configuration/RConn1 -- Ideal Heat Flow Source/RConn2
  C In/RConn1 -- Pressure & Temperature Sensor (TL)2/LConn1 -- Pressure & Temperature Sensor (TL)/LConn1 -- Coldplate/LConn1
  Thermal Reference1/LConn1 -- Ideal Temperature Sensor/RConn1
  Ideal Temperature Sensor/RConn2 -- PS-Simulink Converter2/LConn1
  PS-Simulink Converter3/LConn1 -- Pressure & Temperature Sensor (TL)2/RConn2
  PS-Simulink Converter1/LConn1 -- Pressure & Temperature Sensor (TL)/RConn1

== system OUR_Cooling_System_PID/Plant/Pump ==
  U_pump : Inport
  Coolant : Subsystem
  Pump Control Unit : Subsystem
  To Workspace : ToWorkspace  VariableName=Pump_Press_Out  SaveFormat=Timeseries  SampleTime=-1
  " C_In" : PMIOPort  Side=Left
  C_Out : PMIOPort  Port=2  Side=Right
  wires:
  U_pump/1 -> Pump Control Unit/1(U_pump)
  Pump Control Unit/1(omega_pump) -> Coolant/1(Omega Pump [rad/s])  "Omega Pump [rad/s]"
  Coolant/1(dPressure) -> To Workspace/1
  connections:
  " C_In"/RConn1 -- Coolant/RConn2
  C_Out/RConn1 -- Coolant/RConn1

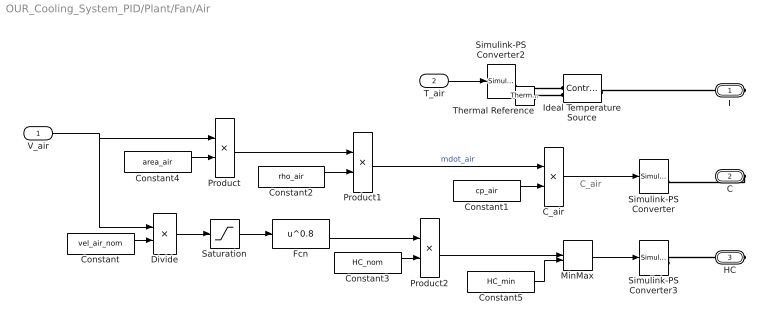
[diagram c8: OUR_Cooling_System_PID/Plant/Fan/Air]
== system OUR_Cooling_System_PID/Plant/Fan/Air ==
  note: C_air
  V_air : Inport
  T_air : Inport  Port=2
  C_air : Product
  Constant : Constant  Value=vel_air_nom
  Constant1 : Constant  Value=cp_air
  Constant2 : Constant  Value=rho_air
  Constant3 : Constant  Value=HC_nom
  Constant4 : Constant  Value=area_air
  Constant5 : Constant  Value=HC_min
  Divide : Product  Inputs=*/
  Fcn : Fcn  Expr=u^0.8
  Ideal Temperature Source : fl_lib/Thermal/Thermal Sources/Controlled Temperature Source
  MinMax : MinMax  Function=max  Inputs=2
  Product : Product
  Product1 : Product
  Product2 : Product
  Saturation : Saturate  UpperLimit=inf  LowerLimit=0
  Simulink-PS Converter : nesl_utility/Simulink-PS Converter  PhysicalDomain=network_engine_domain  SubClassName=ps_input  LeftPortType=input  RightPortType=output  PseudoPeriodic=off  Frequencies=[]  NoiseDistribution=none  NoiseParameters=[]  Unit=W/K  AffineConversion=off  FilteringAndDerivatives=zero  SimscapeFilterOrder=1  InputFilterTimeConstant=1  UdotUserProvided=1
  Simulink-PS Converter2 : nesl_utility/Simulink-PS Converter  PhysicalDomain=network_engine_domain  SubClassName=ps_input  LeftPortType=input  RightPortType=output  PseudoPeriodic=off  Frequencies=[]  NoiseDistribution=none  NoiseParameters=[]  Unit=K  AffineConversion=on  FilteringAndDerivatives=zero  SimscapeFilterOrder=1  InputFilterTimeConstant=1  UdotUserProvided=1
  Simulink-PS Converter3 : nesl_utility/Simulink-PS Converter  PhysicalDomain=network_engine_domain  SubClassName=ps_input  LeftPortType=input  RightPortType=output  PseudoPeriodic=off  Frequencies=[]  NoiseDistribution=none  NoiseParameters=[]  Unit=W/K  AffineConversion=off  FilteringAndDerivatives=zero  SimscapeFilterOrder=1  InputFilterTimeConstant=1  UdotUserProvided=1
  Thermal Reference : fl_lib/Thermal/Thermal Elements/Thermal Reference
  T : PMIOPort  Side=Right
  C : PMIOPort  Port=2  Side=Right
  HC : PMIOPort  Port=3  Side=Right
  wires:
  V_air/1 -> Product/1, Divide/1
  Constant/1 -> Divide/2
  Constant3/1 -> Product2/2
  Divide/1 -> Saturation/1
  Fcn/1 -> Product2/1
  Product2/1 -> MinMax/1
  Constant5/1 -> MinMax/2
  MinMax/1 -> Simulink-PS Converter3/1
  T_air/1 -> Simulink-PS Converter2/1
  Constant1/1 -> C_air/2
  C_air/1 -> Simulink-PS Converter/1
  Product/1 -> Product1/1
  Constant2/1 -> Product1/2
  Constant4/1 -> Product/2
  Product1/1 -> C_air/1  "mdot_air"
  Saturation/1 -> Fcn/1
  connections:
  C/RConn1 -- Simulink-PS Converter/RConn1
  Simulink-PS Converter3/RConn1 -- HC/RConn1
  Thermal Reference/LConn1 -- Ideal Temperature Source/RConn2
  Simulink-PS Converter2/RConn1 -- Ideal Temperature Source/RConn1
  Ideal Temperature Source/LConn1 -- T/RConn1

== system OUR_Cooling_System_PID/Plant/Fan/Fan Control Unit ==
  Veh_speed : Inport
  U_fan : Inport  Port=2
  Subsystem : Subsystem
  V_air (m/s) : Outport  VectorParamsAs1DForOutWhenUnconnected=off
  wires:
  Veh_speed/1 -> Subsystem/1(Veh_speed)
  U_fan/1 -> Subsystem/2(U_fan)
  Subsystem/1(V_air (m/s)) -> V_air (m/s)/1

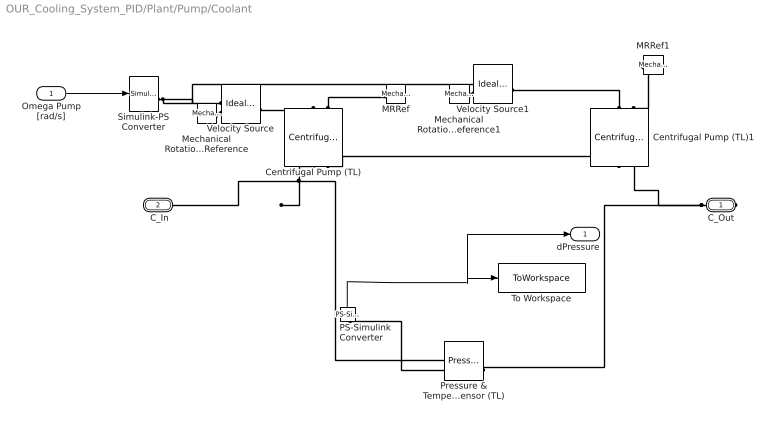
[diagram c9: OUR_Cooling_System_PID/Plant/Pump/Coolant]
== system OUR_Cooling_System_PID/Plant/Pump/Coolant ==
  Omega Pump [rad/s] : Inport
  Centrifugal Pump (TL) : SimscapeFluids_lib/Thermal Liquid/Pumps & Motors/Centrifugal Pump (TL)  pump_parameterization=fluids.thermal_liquid.pumps_motors.enum.CentrifugalPumpParameterization.Nominal  capacity_ref_nominal=15 lpm  head_ref_nominal=1.3 m  power_ref_nominal=0.85 kW  head_ref_max=2.4 m  capacity_ref_max=22.7 lpm  omega_ref_analytic=3000 rpm  flow_rate_1D_TLU=[16.67, 30, 40, 53.33, 66.67, 83.33] lpm  head_1D_TLU=[50, 47.5, 45, 40, 35, 25] m  power_1D_TLU=[.6, .75, .85, .93, .98, .99] kW  omega_ref_1D=3500 rpm  rho_ref_1D=998.21 kg/m^3  omega_threshold_factor=1e-2  flow_rate_2D_TLU=[16.67, 23.33, 30, 40, 53.33, 60] lpm  omega_2D_TLU=[2450, 2800, 3150, 3500] rpm  head_2D_TLU=[25, 32.7, 42.5, 50; 24, 31.7, 41, 49; 22.7, 30.5, 39, 47.5; 20, 28, 36, 45; 15.7, 24, 32, 40; 12.5, 21, 29.5, 37.5] m  power_2D_TLU=[.28, .38, .5, .6; .31, .41, .55, .68; .33, .44, .6, .75; .36, .48, .65, .83; .38, .53, .72, .93; .39, .55, .75, .97] kW  rho_ref_2D=998.21 kg/m^3  diameter_ratio=1  mech_orientation=fluids.thermal_liquid.pumps_motors.enum.CentrifugalPumpMechOrientation.Positive  area=0.005 m^2  operation_check=simscape.enum.assert.action.none
  Centrifugal Pump (TL)1 : SimscapeFluids_lib/Thermal Liquid/Pumps & Motors/Centrifugal Pump (TL)  pump_parameterization=fluids.thermal_liquid.pumps_motors.enum.CentrifugalPumpParameterization.Nominal  capacity_ref_nominal=15 lpm  head_ref_nominal=1.3 m  power_ref_nominal=0.85 kW  head_ref_max=2.4 m  capacity_ref_max=22.7 lpm  omega_ref_analytic=3000 rpm  flow_rate_1D_TLU=[16.67, 30, 40, 53.33, 66.67, 83.33] lpm  head_1D_TLU=[50, 47.5, 45, 40, 35, 25] m  power_1D_TLU=[.6, .75, .85, .93, .98, .99] kW  omega_ref_1D=3500 rpm  rho_ref_1D=998.21 kg/m^3  omega_threshold_factor=1e-2  flow_rate_2D_TLU=[16.67, 23.33, 30, 40, 53.33, 60] lpm  omega_2D_TLU=[2450, 2800, 3150, 3500] rpm  head_2D_TLU=[25, 32.7, 42.5, 50; 24, 31.7, 41, 49; 22.7, 30.5, 39, 47.5; 20, 28, 36, 45; 15.7, 24, 32, 40; 12.5, 21, 29.5, 37.5] m  power_2D_TLU=[.28, .38, .5, .6; .31, .41, .55, .68; .33, .44, .6, .75; .36, .48, .65, .83; .38, .53, .72, .93; .39, .55, .75, .97] kW  rho_ref_2D=998.21 kg/m^3  diameter_ratio=1  mech_orientation=fluids.thermal_liquid.pumps_motors.enum.CentrifugalPumpMechOrientation.Positive  area=0.005 m^2  operation_check=simscape.enum.assert.action.none
  MRRef : fl_lib/Mechanical/Rotational Elements/Mechanical Rotational Reference
  MRRef1 : fl_lib/Mechanical/Rotational Elements/Mechanical Rotational Reference
  Mechanical Rotational Reference : fl_lib/Mechanical/Rotational Elements/Mechanical Rotational Reference
  Mechanical Rotational Reference1 : fl_lib/Mechanical/Rotational Elements/Mechanical Rotational Reference
  PS-Simulink Converter : nesl_utility/PS-Simulink Converter  PhysicalDomain=network_engine_domain  SubClassName=ps_output  LeftPortType=input  RightPortType=output  PseudoPeriodic=off  Frequencies=[]  VectorFormat=inherit  Unit=inherit  AffineConversion=off
  Pressure & Temperature Sensor (TL) : fl_lib/Thermal Liquid/Sensors/Pressure & Temperature Sensor (TL)  reference=foundation.enum.MeasurementReference.difference  pressure=true  pressure_spec=foundation.enum.PressureMeasementSpec.Absolute  temperature=false
  Simulink-PS Converter : nesl_utility/Simulink-PS Converter  PhysicalDomain=network_engine_domain  SubClassName=ps_input  LeftPortType=input  RightPortType=output  PseudoPeriodic=off  Frequencies=[]  NoiseDistribution=none  NoiseParameters=[]  Unit=rad/s  AffineConversion=off  FilteringAndDerivatives=zero  SimscapeFilterOrder=1  InputFilterTimeConstant=0.001  UdotUserProvided=1
  To Workspace : ToWorkspace  VariableName=delta_Pressure  SaveFormat=Timeseries  SampleTime=-1
  Velocity Source : fl_lib/Mechanical/Mechanical Sources/Ideal Angular Velocity Source
  Velocity Source1 : fl_lib/Mechanical/Mechanical Sources/Ideal Angular Velocity Source
  C_Out : PMIOPort  Side=Right
  " C_In" : PMIOPort  Port=2  Side=Right
  dPressure : Outport
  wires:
  PS-Simulink Converter/1 -> dPressure/1, To Workspace/1
  Omega Pump [rad/s]/1 -> Simulink-PS Converter/1
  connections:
  Centrifugal Pump (TL)/LConn1 -- Pressure & Temperature Sensor (TL)/RConn1 -- " C_In"/RConn1
  Centrifugal Pump (TL)/RConn1 -- Velocity Source/LConn1
  Simulink-PS Converter/RConn1 -- Velocity Source1/RConn1 -- Velocity Source/RConn1
  Centrifugal Pump (TL)/RConn2 -- MRRef/LConn1
  Centrifugal Pump (TL)1/LConn1 -- Centrifugal Pump (TL)/LConn2
  Mechanical Rotational Reference/LConn1 -- Velocity Source/RConn2
  C_Out/RConn1 -- Pressure & Temperature Sensor (TL)/LConn1 -- Centrifugal Pump (TL)1/LConn2
  Pressure & Temperature Sensor (TL)/RConn2 -- PS-Simulink Converter/LConn1
  Centrifugal Pump (TL)1/RConn1 -- Velocity Source1/LConn1
  MRRef1/LConn1 -- Centrifugal Pump (TL)1/RConn2
  Mechanical Rotational Reference1/LConn1 -- Velocity Source1/RConn2

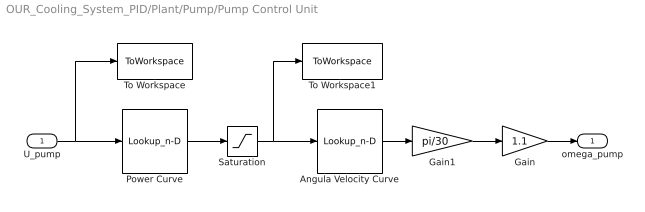
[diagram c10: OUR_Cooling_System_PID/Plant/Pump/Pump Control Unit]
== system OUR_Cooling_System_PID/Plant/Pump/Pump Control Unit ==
  U_pump : Inport
  Angula Velocity Curve : Lookup_n-D  NumberOfTableDimensions=1  BreakpointsForDimension1=[0,100]  Table=[50,3000]  InternalRulePriority=Speed  RndMeth=Simplest
  Gain : Gain  Gain=1.1
  Gain1 : Gain  Gain=pi/30
  Power Curve : Lookup_n-D  NumberOfTableDimensions=1  BreakpointsForDimension1=[0,100]  Table=[0,P_nom_pump]  InternalRulePriority=Speed  RndMeth=Simplest
  Saturation : Saturate  UpperLimit=14.4  LowerLimit=0
  To Workspace : ToWorkspace  VariableName=Pump_DC  SaveFormat=Timeseries  SampleTime=-1
  To Workspace1 : ToWorkspace  VariableName=Pump_Power  SaveFormat=Timeseries  SampleTime=-1
  omega_pump : Outport
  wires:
  Saturation/1 -> To Workspace1/1, Angula Velocity Curve/1
  Gain/1 -> omega_pump/1
  Gain1/1 -> Gain/1
  Angula Velocity Curve/1 -> Gain1/1
  U_pump/1 -> To Workspace/1, Power Curve/1
  Power Curve/1 -> Saturation/1

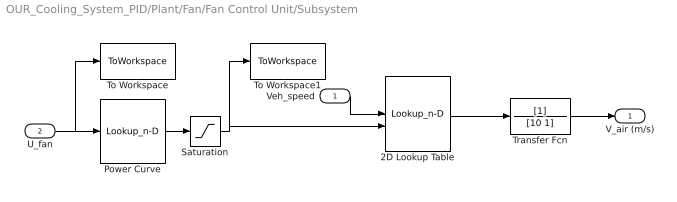
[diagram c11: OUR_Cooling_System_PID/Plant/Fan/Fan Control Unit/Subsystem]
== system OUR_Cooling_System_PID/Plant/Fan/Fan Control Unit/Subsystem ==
  Veh_speed : Inport
  U_fan : Inport  Port=2
  2D Lookup Table : Lookup_n-D  LookupTableObject=''  BreakpointsForDimension1=[0 10 30 50 75 100]  BreakpointsForDimension2=[0 3.6 7.2 10.8 14.4]  Table=[0 7 13 19 25;2.4 9 16 24 32;7.2 14 20 29 39;11.4 17 23 34 45;18.8 23 25 37 49;23 24 26 39 51]  InternalRulePriority=Speed  RndMeth=Simplest
  Power Curve : Lookup_n-D  NumberOfTableDimensions=1  BreakpointsForDimension1=[0,14.4]  Table=[50,3000]  InternalRulePriority=Speed  RndMeth=Simplest
  Saturation : Saturate
  To Workspace : ToWorkspace  VariableName=Fan_DC  SaveFormat=Timeseries  SampleTime=-1
  To Workspace1 : ToWorkspace  VariableName=Fan_Power  SaveFormat=Timeseries  SampleTime=-1
  Transfer Fcn : TransferFcn  Denominator=[10 1]
  V_air (m/s) : Outport  VectorParamsAs1DForOutWhenUnconnected=off
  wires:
  Transfer Fcn/1 -> V_air (m/s)/1
  2D Lookup Table/1 -> Transfer Fcn/1
  Veh_speed/1 -> 2D Lookup Table/1
  U_fan/1 -> To Workspace/1, Power Curve/1
  Saturation/1 -> To Workspace1/1, 2D Lookup Table/2
  Power Curve/1 -> Saturation/1
